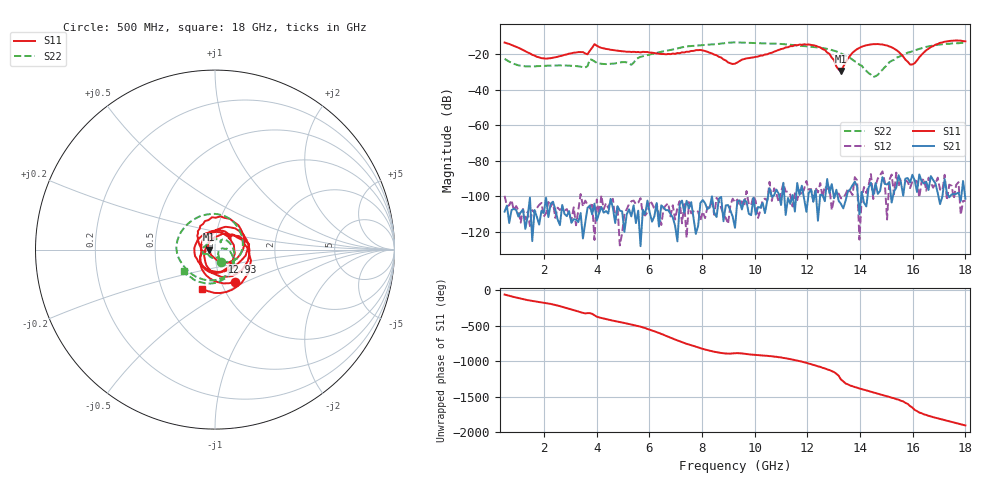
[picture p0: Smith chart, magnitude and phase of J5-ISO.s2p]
!Agilent Technologies,N5230C,MY49001096,A.09.42.15
!Agilent N5230C: A.09.42.15
!Date: Thursday, June 29, 2023 08:14:40
!Correction: S11(Full 2 Port(1,2))
!S21(Full 2 Port(1,2))
!S12(Full 2 Port(1,2))
!S22(Full 2 Port(1,2))
!S2P File: Measurements: S11, S21, S12, S22:
# Hz S  dB  R 50
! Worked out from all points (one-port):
!   201 points, 500 MHz to 18 GHz, reference 50 ohm
!   lowest |S11| = -29.5 dB at 13.28 GHz (marker M1), VSWR 1.07, Z = 46.8 - j0.0267 ohm
!   |S11| at or under -10 dB: start of sweep to end of sweep
!   S11 on the Smith chart (normalised r, x): 500 MHz: 1.17, -0.44; 12.93 GHz: 1.07, -0.15; 18 GHz: 0.79, -0.37
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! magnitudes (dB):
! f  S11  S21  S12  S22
! 500 MHz  -13.4  -108.7  -99.8  -22.6
! 1.025 GHz  -16.3  -111.5  -107.9  -26.2
! 1.9 GHz  -22.2  -108.3  -103.8  -26.6
! 3.475 GHz  -18.8  -123.8  -105.8  -27.3
! 3.65 GHz  -20.0  -106.5  -104.9  -26.7
! 3.737 GHz  -18.0  -105.2  -106.8  -22.8
! 3.913 GHz  -14.3  -104.2  -124.6  -24.0
! 5.312 GHz  -18.8  -111.4  -102.9  -26.0
! 5.575 GHz  -18.7  -108.2  -103.6  -22.1
! 6.362 GHz  -19.7  -117.1  -110.8  -18.9
! 7.938 GHz  -17.6  -103.8  -113.5  -15.0
! 9.25 GHz  -25.3  -117.8  -103.6  -13.3
! 11.35 GHz  -15.4  -104.3  -99.1  -14.6
! 12.22 GHz  -15.0  -103.1  -103.0  -15.9
! 12.93 GHz  -21.9  -93.2  -107.8  -17.6
! 13.28 GHz  -29.5  -104.4  -101.2  -19.5
! 13.8 GHz  -18.1  -91.8  -89.3  -24.0
! 14.5 GHz  -14.3  -99.3  -101.6  -32.9
! 15.11 GHz  -15.6  -92.0  -90.9  -24.5
! 15.99 GHz  -25.8  -87.9  -91.5  -18.3
! 16.86 GHz  -14.6  -92.8  -92.9  -14.9
! 18 GHz  -12.7  -101.4  -102.6  -13.5
